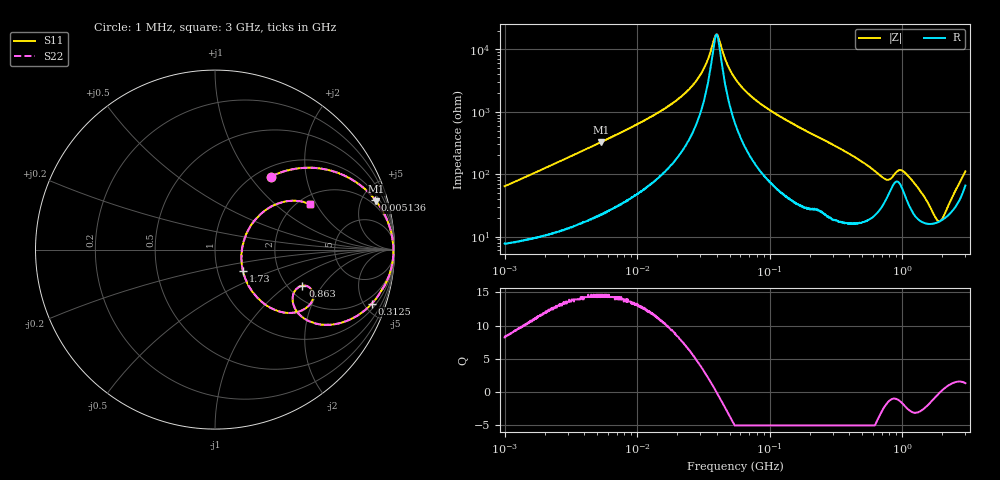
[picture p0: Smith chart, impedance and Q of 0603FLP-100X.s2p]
!s-Parameter Generated by FASTRON Sdn. Bhd.
!FASTRON P/N : 0603FLP-100X
!Keysight Technologies: E4991B_MY54100416_A.01.15
!Date: Tue Dec 02 13:12:42 2025
!Version  :Rev00  Tue Dec 02 13:12:42 2025
!Data & Calibration Information:
!Freq  S11  S21  S12  S22
!PortZ  Port1:50+j0  Port2:50+j0
!When reading reference impedance value at option line is always used.
! Remarks : This data is being provided solely for informational purposes.
# Hz S dB R 50
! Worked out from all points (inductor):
!   1601 points, 1 MHz to 3 GHz, reference 50 ohm
!   read as one part in series: L = 9.96 uH near 1.041 MHz
!   highest Q = 14.7 at 5.373 MHz (marker M1), where L = 9.73 uH
!   self-resonance near 39.56 MHz
!   S11 on the Smith chart (normalised r, x): 1 MHz: 1.15, +1.27; 5.136 MHz: 1.43, +6.25; 312.5 MHz: 1.37, -5.65; 863 MHz: 2.38, -1.33; 1.73 GHz: 1.32, -0.32; 3 GHz: 2.32, +1.78
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1000000  -5.81 52.5  -1.95 -30.6  -1.95 -30.6  -5.81 52.5
1869176  -2.77 38.6  -4.06 -46.4  -4.06 -46.4  -2.77 38.6
3804036  -0.95 22.6  -8.28 -63.4  -8.28 -63.4  -0.95 22.6
5136138  -0.59 17.3  -10.50 -68.7  -10.50 -68.7  -0.59 17.3
5372736  -0.55 16.6  -10.90 -69.5  -10.90 -69.5  -0.55 16.6
1.447069e7  -0.12 5.8  -19.90 -79.1  -19.90 -79.1  -0.12 5.8
2.745737e7  -0.06 1.9  -29.50 -77.0  -29.50 -77.0  -0.06 1.9
3.287715e7  -0.05 0.9  -35.10 -69.0  -35.10 -69.0  -0.05 0.9
3.956422e7  -0.05 0.0  -44.80 -4.1  -44.80 -4.1  -0.05 0.0
5.504702e7  -0.05 -1.7  -30.60 77.5  -30.60 77.5  -0.05 -1.7
8.593077e7  -0.08 -4.3  -22.50 81.1  -22.50 81.1  -0.08 -4.3
2.083556e8  -0.34 -12.6  -13.20 73.8  -13.20 73.8  -0.34 -12.6
3.124888e8  -0.68 -19.0  -9.71 67.3  -9.71 67.3  -0.68 -19.0
5.7828e8  -2.71 -34.8  -4.76 46.4  -4.76 46.4  -2.71 -34.8
7.925923e8  -5.98 -29.8  -4.20 23.9  -4.20 23.9  -5.98 -29.8
8.629671e8  -5.56 -22.4  -5.18 21.4  -5.18 21.4  -5.56 -22.4
9.977393e8  -4.28 -27.1  -5.44 31.4  -5.44 31.4  -4.28 -27.1
1.200675e9  -5.41 -41.1  -3.19 30.6  -3.19 30.6  -5.41 -41.1
1.730092e9  -14.20 -37.2  -1.38 8.0  -1.38 8.0  -14.20 -37.2
1.970482e9  -16.20 7.3  -1.45 -1.3  -1.45 -1.3  -16.20 7.3
2.530652e9  -7.99 37.4  -2.80 -19.5  -2.80 -19.5  -7.99 37.4
3e9  -4.61 25.3  -5.49 -28.2  -5.49 -28.2  -4.61 25.3
